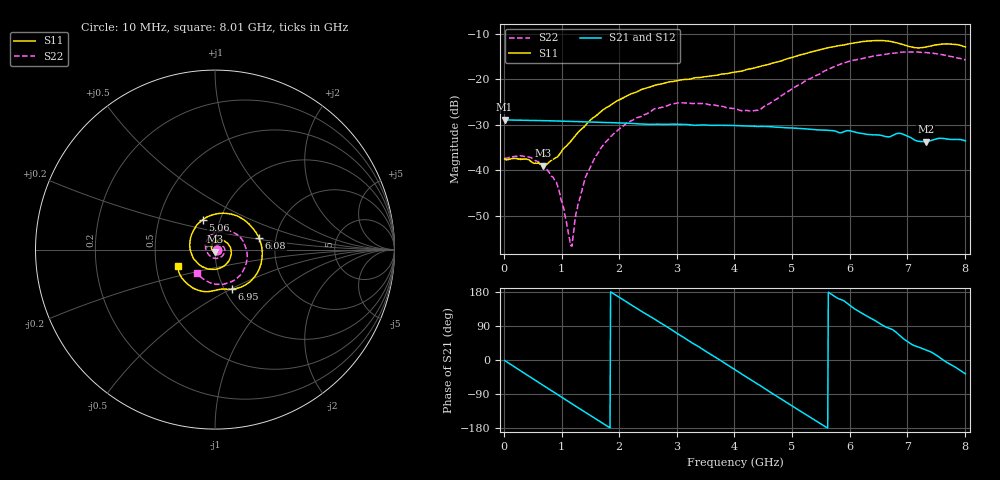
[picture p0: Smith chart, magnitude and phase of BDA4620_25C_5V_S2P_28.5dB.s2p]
!Agilent Technologies,E5071B,MY42404982,A.09.10
!Date: Wed May 06 09:04:40 2026
!Data & Calibration Information:
!Freq	S11:SOLT2(ON)	S21:SOLT2(ON)	S12:SOLT2(ON)	S22:SOLT2(ON)
# Hz S RI R 50
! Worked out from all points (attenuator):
!   801 points, 10 MHz to 8.01 GHz, reference 50 ohm
!   highest |S21| = -28.88 dB at 10 MHz (marker M1); lowest = -33.7 dB at 7.32 GHz (marker M2)
!   lowest |S11| = -39.0 dB at 680 MHz (marker M3), VSWR 1.02, Z = 49.8 - j1.1 ohm
!   |S11| at or under -10 dB: start of sweep to end of sweep
!   |S22| runs from -56.7 to -13.9 dB; largest |S21 - S12| = 0.00019
!   S11 on the Smith chart (normalised r, x): 10 MHz: 1.03, -0.00; 5.06 GHz: 0.83, +0.28; 6.08 GHz: 1.63, +0.23; 6.95 GHz: 1.08, -0.51; 8.01 GHz: 0.65, -0.13
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1e7  0.0133 -0.000823  0.036 -0.000703  0.036 -0.000771  0.0134 -0.000437
4.1e8  0.00822 -0.0102  0.0269 -0.023  0.027 -0.0231  0.0133 -0.00456
6.8e8  -0.00199 -0.011  0.0138 -0.0324  0.0138 -0.0324  0.00919 -0.0065
9.3e8  -0.0132 -0.0049  -0.000793 -0.0349  -0.000838 -0.0349  0.00359 -0.00571
1.16e9  -0.0194 0.00772  -0.0139 -0.0316  -0.0139 -0.0317  -0.00127 -0.000755
1.19e9  -0.0199 0.00975  -0.0154 -0.0308  -0.0155 -0.0308  -0.0017 0.000146
1.35e9  -0.0195 0.0209  -0.023 -0.0254  -0.023 -0.0254  -0.00317 0.00497
1.53e9  -0.0138 0.0343  -0.0292 -0.0173  -0.0292 -0.0173  -0.00297 0.0115
1.77e9  0.00235 0.0484  -0.0333 -0.00447  -0.0333 -0.00443  0.00119 0.0205
2.15e9  0.0421 0.0517  -0.0288 0.0159  -0.0289 0.016  0.0174 0.0289
2.68e9  0.0882 0.00402  -0.00632 0.0315  -0.00632 0.0315  0.0442 0.0191
3.08e9  0.0802 -0.0583  0.0144 0.0285  0.0145 0.0285  0.055 -0.00764
4.01e9  -0.083 -0.0877  0.028 -0.0135  0.028 -0.0135  -0.0106 -0.0463
4.42e9  -0.138 -0.000885  0.0128 -0.0275  0.0129 -0.0276  -0.0446 -0.0124
5.06e9  -0.0694 0.1656  -0.0174 -0.0233  -0.0175 -0.0233  -0.0237 0.0798
5.35e9  0.0217 0.2016  -0.0254 -0.0121  -0.0255 -0.0121  0.0233 0.1021
6.08e9  0.2443 0.0668  -0.0189 0.0185  -0.0189 0.0185  0.157 0.0453
6.68e9  0.1927 -0.181  0.00242 0.0232  0.0024 0.0232  0.1696 -0.09
6.95e9  0.0941 -0.2204  0.0143 0.0199  0.0143 0.02  0.1346 -0.1482
7.32e9  0.00229 -0.2277  0.0184 0.00929  0.0184 0.00931  0.0491 -0.192
7.65e9  -0.1176 -0.2169  0.0223 -0.00107  0.0223 -0.00104  -0.0328 -0.1824
8.01e9  -0.2086 -0.0925  0.0169 -0.0125  0.0171 -0.0125  -0.1025 -0.1283
